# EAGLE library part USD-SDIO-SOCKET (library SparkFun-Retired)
microSD Socket Push-push type uSD socket with full SDIO signal mapping. Spark Fun Electronics SKU : PRT-00127. tDoc lines correctly indicate media card edge positions when inserting (unlocked, locked, depressed). NOTE: CD1 and CD2 are connected internally, and short to ground when card is removed.
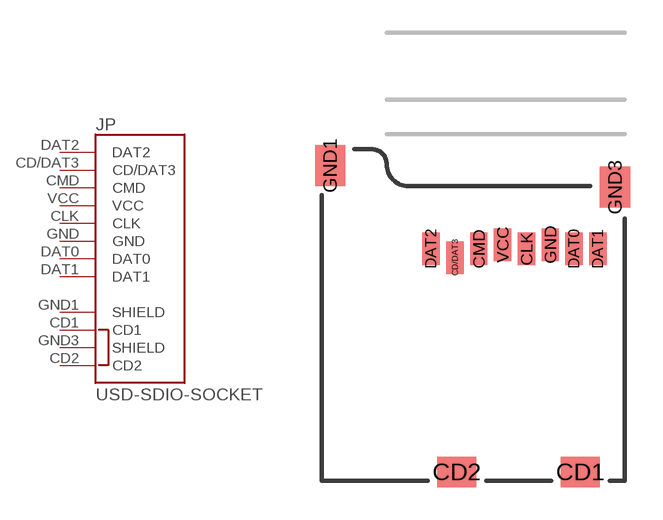
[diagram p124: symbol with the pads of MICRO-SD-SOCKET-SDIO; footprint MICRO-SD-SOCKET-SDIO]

Designator prefix JP

## USD-SDIO-SOCKET (PROD_ID: CONN-07820)  [MICRO-SD-SOCKET-SDIO]
CD1  CD1
CD2  CD2
CD/DAT3  CD/DAT3
CLK  CLK
CMD  CMD
DAT0  DAT0
DAT1  DAT1
DAT2  DAT2
GND  GND
GND1  SHIELD
GND3  SHIELD
VCC  VCC

## Footprint MICRO-SD-SOCKET-SDIO (pad centres in mm)
smd 1.8 x 1.4: CD1 11.92,0.4; CD2 6.22,0.4
smd 0.8 x 1.5: CD/DAT3 6.13,10.3; CLK 9.43,10.7; CMD 7.23,10.7; DAT0 11.63,10.7; DAT1 12.73,10.7; DAT2 5.03,10.7; GND 10.53,10.9; VCC 8.33,10.9
smd 1.4 x 1.9: GND1 0.37,14.55; GND3 13.52,13.55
